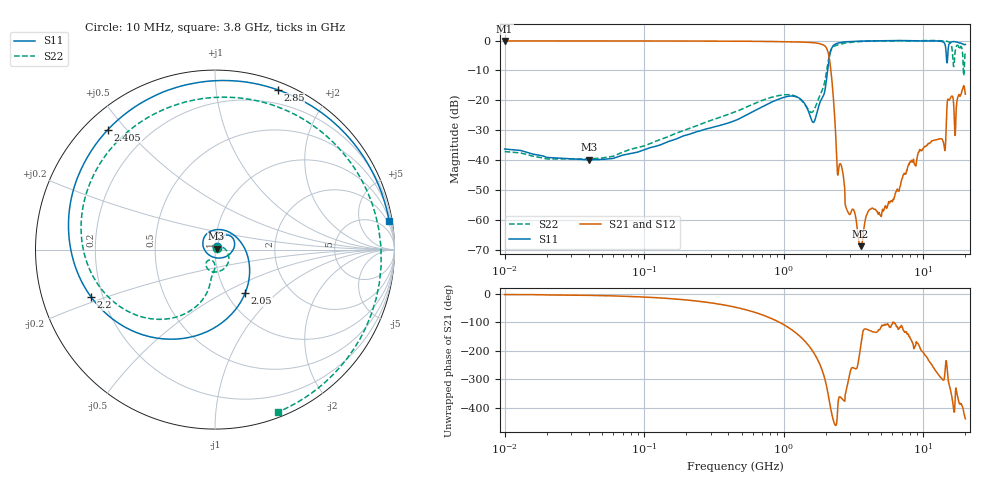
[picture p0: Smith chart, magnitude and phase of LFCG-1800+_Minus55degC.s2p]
! Mini-Circuits
! S2P DATA File Format
! Type: LOW PASS FILTER
! Model: LFCG-1800+
! All S Parameters are in dB deg format
! TEST CONDITIONS: INPUT POWER = 0 dBm @ Temperature = -55deg C
!S2P File: Measurements: S11, S21, S12, S22:
# Hz S  dB  R 50
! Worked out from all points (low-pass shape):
!   718 points, 10 MHz to 20 GHz, reference 50 ohm
!   highest |S21| = -0.10 dB at 10 MHz (marker M1); lowest = -68.7 dB at 3.55 GHz (marker M2)
!   |S21| within 3 dB of the highest: start of sweep to 2.05 GHz
!   lowest |S11| = -39.9 dB at 40 MHz (marker M3), VSWR 1.02, Z = 50.9 + j0.501 ohm
!   |S11| at or under -10 dB: start of sweep to 2.057 GHz
!   |S22| runs from -39.6 to 0.0 dB; largest |S21 - S12| = 0.0012
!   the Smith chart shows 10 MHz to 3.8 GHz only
!   S11 on the Smith chart (normalised r, x): 10 MHz: 1.02, +0.02; 2.05 GHz: 1.22, -0.65; 2.2 GHz: 0.16, -0.18; 2.405 GHz: 0.07, +0.45; 2.85 GHz: 0.07, +1.46; 3.8 GHz: 1, +12
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1e7  -36.26 52.3  -0.10 -1.5  -0.10 -1.6  -37.11 51.6
4e7  -39.87 29.0  -0.11 -4.4  -0.11 -4.4  -39.57 27.4
1.3e8  -34.91 48.7  -0.14 -13.5  -0.13 -13.5  -33.13 31.8
4.5e8  -26.69 65.5  -0.21 -46.2  -0.21 -46.2  -23.79 -6.0
1.02e9  -18.89 42.4  -0.39 -110.2  -0.39 -110.2  -18.08 -84.5
1.59e9  -26.82 -86.3  -0.67 163.3  -0.67 163.3  -24.02 -106.6
1.875e9  -19.37 96.9  -1.26 94.3  -1.25 94.2  -16.82 -96.0
2.05e9  -10.60 -55.3  -3.11 22.6  -3.10 22.6  -8.75 -111.8
2.2e9  -2.63 -159.0  -12.25 -59.0  -12.24 -59.0  -2.71 -179.2
2.405e9  -0.95 131.8  -41.58 -83.7  -41.58 -83.7  -1.54 102.3
2.85e9  -0.38 68.6  -56.87 38.0  -56.89 38.2  -0.73 6.9
3.55e9  -0.18 20.9  -68.73 172.9  -68.82 173.3  -0.32 -56.2
3.8e9  -0.15 9.3  -60.99 -123.0  -60.96 -122.9  -0.26 -68.9
5.65e9  -0.02 -38.2  -53.83 -109.4  -53.80 -109.4  -0.06 -117.5
9.15e9  -0.10 -77.5  -37.87 -173.7  -37.90 -173.8  -0.08 179.5
1.215e10  -0.09 -110.8  -33.26 92.1  -33.26 92.1  0.01 119.6
1.425e10  -1.12 -174.0  -36.75 80.3  -36.74 80.2  -0.11 85.2
1.6e10  -0.41 156.8  -18.57 -1.8  -18.56 -2.0  -2.38 30.4
1.645e10  -0.34 146.0  -20.89 -43.6  -20.89 -43.7  -8.61 -80.1
1.685e10  -0.39 138.9  -31.74 -20.3  -31.70 -20.3  -4.10 158.5
1.91e10  -1.11 125.6  -16.28 -38.1  -16.29 -38.3  -4.39 67.1
2e10  -1.31 116.4  -17.93 -79.2  -17.89 -79.4  -3.89 114.1
